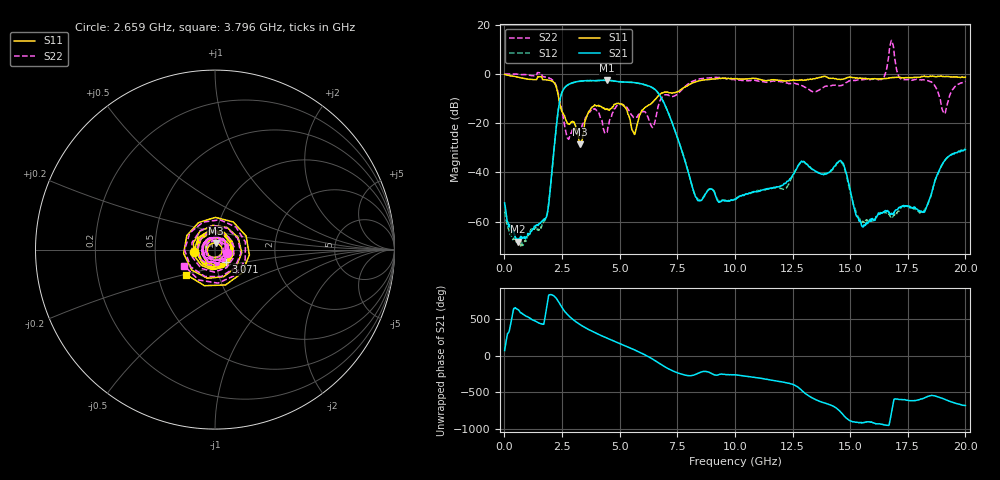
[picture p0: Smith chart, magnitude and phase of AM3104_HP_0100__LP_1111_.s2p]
!Created with skrf (http://scikit-rf.org).
# Hz S RI R 50.0
!freq ReS11 ImS11 ReS21 ImS21 ReS12 ImS12 ReS22 ImS22
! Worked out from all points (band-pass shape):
!   1601 points, 10 MHz to 20 GHz, reference 50 ohm
!   highest |S21| = -2.58 dB at 4.458 GHz (marker M1); lowest = -68.1 dB at 597.2 MHz (marker M2)
!   |S21| within 3 dB of the highest: 2.617 GHz to 6.424 GHz (3.807 GHz wide, 84.2 % of centre)
!   lowest |S11| = -28.6 dB at 3.283 GHz (marker M3), VSWR 1.08, Z = 50.3 + j3.72 ohm
!   |S11| at or under -10 dB: 2.358 GHz to 6.577 GHz (4.219 GHz wide, 94.4 % of centre)
!   |S22| runs from -26.6 to 13.6 dB; largest |S21 - S12| = 0.083
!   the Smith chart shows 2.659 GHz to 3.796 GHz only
!   S11 on the Smith chart (normalised r, x): 2.659 GHz: 0.79, -0.02; 3.071 GHz: 1.12, -0.15; 3.796 GHz: 0.70, -0.20
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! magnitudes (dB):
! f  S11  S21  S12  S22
! 10 MHz  -0.2  -52.4  -55.9  0.0
! 597.2 MHz  -1.3  -68.1  -68.3  -0.1
! 1.822 GHz  -2.4  -58.3  -57.9  -1.3
! 2.359 GHz  -10.0  -13.4  -13.4  -8.9
! 2.659 GHz  -18.5  -5.1  -5.1  -23.2
! 3.071 GHz  -20.8  -3.3  -3.3  -22.7
! 3.283 GHz  -28.6  -2.9  -3.0  -22.7
! 3.346 GHz  -27.4  -2.8  -2.9  -22.0
! 3.796 GHz  -13.5  -2.7  -2.8  -14.3
! 4.458 GHz  -14.3  -2.6  -2.6  -23.7
! 4.958 GHz  -11.9  -3.1  -3.2  -12.4
! 5.62 GHz  -24.1  -3.5  -3.5  -17.7
! 6.682 GHz  -8.8  -7.8  -7.8  -12.9
! 8.356 GHz  -3.1  -50.9  -50.5  -2.3
! 10.01 GHz  -2.0  -51.1  -50.8  -2.4
! 13.34 GHz  -2.2  -38.7  -38.6  -7.1
! 14.64 GHz  -2.2  -35.7  -36.2  -4.7
! 15.56 GHz  -1.8  -62.2  -60.2  -2.3
! 16.68 GHz  -1.7  -56.0  -57.0  7.3
! 18.2 GHz  -0.9  -56.0  -55.6  -2.4
! 19.06 GHz  -1.0  -35.7  -35.7  -15.7
! 20 GHz  -1.3  -30.8  -30.3  -3.0
